| z32d_ut.ibs * IBIS 5.0 Model
| 16Gb DDR4 SDRAM - Die Revision "E"
| This Model is valid for Ultra-High Automotive Temperature Range -40C<=Tc<=125C
| Valid for DDR4-1600/1866/2133/2400/2666/2933/3200 operation
| Models *_3200 are applicable for speed grade 3200 Mbps (-062) and below
| Part Number   VDD/VDDQ   Architecture   Package
| MT40A4G4JE   1.2V/1.2V   4Gb   x  4   78-Ball FBGA
| MT40A2G8JE   1.2V/1.2V   2Gb   x  8   78-Ball FBGA
| MT40A1G16KH   1.2V/1.2V   1Gb   x 16   96-Ball FBGA
| MT40A4G4Z32D   1.2V/1.2V   4Gb   x 4   (Bare Die, x4)
| MT40A2G8Z32D   1.2V/1.2V   2Gb   x 8   (Bare Die, x8)
| MT40A1G16Z32D   1.2V/1.2V   1Gb   x 16   (Bare Die, x16)
[IBIS Ver]   5.0
[File Name]   z32d_ut.ibs
[Date]   5/19/2021
[File Rev]   2.4.2
[Source]   From silicon level SPICE model at Micron Technology, Inc.
   For support contact your local Micron FAE/Sales contacts
   (more information at https://www.micron.com/support/sales-network)
[Notes]   Revision History:
   Rev 2.4.2: 5/19/2021
   - Updated Part Numbers and Package Codes for Automotive parts
   Rev 2.4.1: 11/30/2020
   - Fixed submodels used for ODT models
   Rev 2.4: 11/16/2020
   - Simulated with new device models
   - Added Automotive and Industrial temperature ranges
   Rev 2.3: 9/11/2020
   - Updated c_comp with 8/19/2020 IOCAP measurements
   - Added x16 package model (9/2/2020 data)
   Rev 2.2: 8/4/2020
   - Updated c_comp with 6/25/2020 IOCAP measurements
   - Updated x4 and x8 package configuration based on 7/30/2020 data
   Rev 2.0: 8/27/2019
   - Matched IV curves with 8/22/2019 Z32D silicon measurements
   Rev 0.3: 8/9/2019
   - Component RLC data and Sparse Matrix Package Model updated with
   z32d specific data
   - Added x16 package model.
   Rev 0.2: 8/2/2019
   - Simulations ran with z32d SPF netlists.
   - C_comp values updated with 5/6/2019 z32d iocap data.
   - PU/PD trims similar with z22a trims.
   - Component RLC data and Sparse Matrix Package Model borrowed from z23c.
   - Will get z32d specific trims and package data in a couple of weeks.
   Rev 0.1: 5/17/2019
   - Initial pre-silicon model
   - All models were created from z32c SPF netlists.
   Notes:
   - The DQ_IN_ODT* models contain assumed input thresholds,
   the actual threshold values will depend on the VREFDQ
   level set by training
   - This IBIS file uses the Submodel keyword to model the
   DDR4 On-die Termination(ODT) characteristics.
   - The C_comp value in the DQ I/O model is set to match the
   input state of the DQ I/O as measured from the HSPICE model.
   The C_comp value decreases in the DQ/DQS Input ODT models.
   - L_pin values in the Pin sections are loop inductance and
   include the mutual inductance to appropriate POWER/GND
   return paths.  POWER/GND parasitics are modeled in the
   Package Models.
   - Typ and slow corner V-t curves in the following DQ* models
   are shifted relative to strong corner V-t curve
   to contain all 3 corners within appropriate V-t window
   Models   Typ   Slow   V-t duration
   DQ*_34_3200   -100ps   -240ps   440ps
   DQ*_40_3200   -100ps   -240ps   440ps
   DQ*_48_3200   -100ps   -240ps   440ps
   ALERT_3200   -40ps   -100ps   500ps
   - Due to the shift in typ and slow corner, the V-t curves
   may overlap each other. This does not effect the accuracy
   of the IBIS data.
   - The NF_INPUT Model is for Non-functioning INPUT pins in the
   x8 package
   - The NF_DQ Model is for Non-functioning DQ pins in the
   x4 package
   See Micron IBIS Model Quality Report and Quality Checklist
   for full IQ details
[Disclaimer]  This software code and all associated documentation, comments
   or other information (collectively "Software") is provided
   "AS IS" without warranty of any kind. MICRON TECHNOLOGY, INC.
   ("MTI") EXPRESSLY DISCLAIMS ALL WARRANTIES EXPRESS OR IMPLIED,
   INCLUDING BUT NOT LIMITED TO, NONINFRINGEMENT OF THIRD PARTY
   RIGHTS, AND ANY IMPLIED WARRANTIES OF MERCHANTABILITY OR
   FITNESS FOR ANY PARTICULAR PURPOSE. MTI DOES NOT WARRANT THAT
   THE SOFTWARE WILL MEET YOUR REQUIREMENTS, OR THAT THE
   OPERATION OF THE SOFTWARE WILL BE UNINTERRUPTED OR ERROR-FREE.
   FURTHERMORE, MTI DOES NOT MAKE ANY REPRESENTATIONS REGARDING
   THE USE OR THE RESULTS OF THE USE OF THE SOFTWARE IN TERMS OF
   ITS CORRECTNESS, ACCURACY, RELIABILITY, OR OTHERWISE. THE
   ENTIRE RISK ARISING OUT OF USE OR PERFORMANCE OF THE SOFTWARE
   REMAINS WITH YOU. IN NO EVENT SHALL MTI, ITS AFFILIATED
   COMPANIES OR THEIR SUPPLIERS BE LIABLE FOR ANY DIRECT,
   INDIRECT, CONSEQUENTIAL, INCIDENTAL, OR SPECIAL DAMAGES
   (INCLUDING, WITHOUT LIMITATION, DAMAGES FOR LOSS OF PROFITS,
   BUSINESS INTERRUPTION, OR LOSS OF INFORMATION) ARISING OUT OF
   YOUR USE OF OR INABILITY TO USE THE SOFTWARE, EVEN IF MTI HAS
   BEEN ADVISED OF THE POSSIBILITY OF SUCH DAMAGES. Because some
   jurisdictions prohibit the exclusion or limitation of
   liability for consequential or incidental damages, the above
   limitation may not apply to you.
[Copyright]   Copyright 2021 Micron Technology, Inc. All rights reserved.
| COMPONENT: MT40A4G4JE (78-Ball FBGA, x4)
[Component]   MT40A4G4JE
[Package Model] z32d_78ball_pkg
[Manufacturer]  Micron Technology,Inc.
[Package]
|   typ   min   max
R_pkg   0.456   0.390   0.524
L_pkg   1.988nH   1.619nH   2.308nH
C_pkg   0.525pF   0.416pF   0.832pF
[Pin]   signal_name   model_name   R_pin   L_pin   C_pin   | TD_pin(ps)   Z_pin
A1   VDD   POWER
A2   VSSQ   GND
A3   NF   NF_DQ   0.489   1.750nH   0.545pF   | 30.894   56.647
A7   NF   NF_DQ   0.511   1.874nH   0.589pF   | 33.231   56.384
A8   VSSQ   GND
A9   VSS   GND
B1   VPP   POWER
B2   VDDQ   POWER
B3   DQS_c   DQS   0.486   1.773nH   0.525pF   | 30.517   58.085
B7   DQ1   DQ   0.501   1.800nH   0.562pF   | 31.820   56.584
B8   VDDQ   POWER
B9   ZQ   NC
C1   VDDQ   POWER
C2   DQ0   DQ   0.474   1.679nH   0.533pF   | 29.920   56.108
C3   DQS_t   DQS   0.476   1.822nH   0.496pF   | 30.052   60.618
C7   VDD   POWER
C8   VSS   GND
C9   VDDQ   POWER
D1   VSS   GND
D2   NC   NC
D3   DQ2   DQ   0.472   1.854nH   0.500pF   | 30.432   60.921
D7   DQ3   DQ   0.507   1.896nH   0.570pF   | 32.871   57.672
D8   NC   NC
D9   VSS   GND
E1   VSSL   GND
E2   VDDQ   POWER
E3   NC   NC
E7   NC   NC
E8   VDDQ   POWER
E9   VSS   GND
F1   VDDL   POWER
F2   NC   NC
F3   ODT   INPUT   0.411   1.925nH   0.513pF   | 31.424   61.251
F7   CK_t   CLKIN   0.443   1.798nH   0.465pF   | 28.925   62.150
F8   CK_c   CLKIN   0.444   1.736nH   0.480pF   | 28.878   60.124
F9   VDD   POWER
G1   VSS   GND
G2   NC   NC
G3   CKE   INPUT   0.409   1.964nH   0.404pF   | 28.176   69.706
G7   CS_n   INPUT   0.431   1.908nH   0.432pF   | 28.718   66.430
G8   NC   NC
G9   TEN   INPUT   0.383   1.791nH   0.817pF   | 38.251   46.825
H1   VDD   POWER
H2   WE_n_A14   INPUT   0.418   2.109nH   0.449pF   | 30.769   68.534
H3   ACT_n   INPUT   0.417   1.961nH   0.401pF   | 28.060   69.898
H7   CAS_n_A15   INPUT   0.424   2.012nH   0.494pF   | 31.537   63.804
H8   RAS_n_A16   INPUT   0.454   2.168nH   0.498pF   | 32.847   66.005
H9   VSS   GND
J1   VREFCA   POWER
J2   BG0   INPUT   0.413   2.000nH   0.463pF   | 30.442   65.692
J3   A10   INPUT   0.419   1.998nH   0.414pF   | 28.764   69.471
J7   A12_BC_n   INPUT   0.445   2.033nH   0.493pF   | 31.668   64.200
J8   BG1   INPUT   0.416   2.015nH   0.444pF   | 29.919   67.359
J9   VDD   POWER
K1   VSS   GND
K2   BA0   INPUT   0.411   1.987nH   0.489pF   | 31.161   63.771
K3   A4   INPUT   0.439   2.097nH   0.466pF   | 31.268   67.077
K7   A3   INPUT   0.464   2.043nH   0.494pF   | 31.777   64.281
K8   BA1   INPUT   0.447   1.943nH   0.510pF   | 31.478   61.723
K9   VSS   GND
L1   RESET_n   INPUT   0.362   1.895nH   0.778pF   | 38.392   49.358
L2   A6   INPUT   0.451   2.165nH   0.503pF   | 33.004   65.598
L3   A0   INPUT   0.424   2.147nH   0.458pF   | 31.371   68.448
L7   A1   INPUT   0.468   2.166nH   0.437pF   | 30.762   70.406
L8   A5   INPUT   0.474   2.194nH   0.528pF   | 34.017   64.487
L9   ALERT_n   ALERT   0.367   1.782nH   0.744pF   | 36.422   48.927
M1   VDD   POWER
M2   A8   INPUT   0.409   2.072nH   0.479pF   | 31.515   65.733
M3   A2   INPUT   0.427   2.141nH   0.444pF   | 30.824   69.466
M7   A9   INPUT   0.470   2.288nH   0.481pF   | 33.168   68.967
M8   A7   INPUT   0.447   2.196nH   0.519pF   | 33.774   65.017
M9   VPP   POWER
N1   VSS   GND
N2   A11   INPUT   0.441   2.192nH   0.480pF   | 32.443   67.581
N3   PARITY   INPUT   0.378   1.641nH   0.470pF   | 27.766   59.114
N7   A17   INPUT   0.407   1.906nH   0.476pF   | 30.114   63.296
N8   A13   INPUT   0.469   2.299nH   0.563pF   | 35.991   63.889
N9   VDD   POWER
|***********************PIN MAPPING*****************************************
[Pin Mapping]   pulldown_ref   pullup_ref   gnd_clamp_ref   power_clamp_ref ext_ref
A1   NC   VDD
A2   VSS   NC
A3   NC   NC   VSS   VDDQ
A7   NC   NC   VSS   VDDQ
A8   VSS   NC
A9   VSS   NC
B1   NC   VPP
B2   NC   VDDQ
B3   VSS   VDDQ   VSS   VDDQ
B7   VSS   VDDQ   VSS   VDDQ
B8   NC   VDDQ
B9   NC   NC
C1   NC   VDDQ
C2   VSS   VDDQ   VSS   VDDQ
C3   VSS   VDDQ   VSS   VDDQ
C7   NC   VDD
C8   VSS   NC
C9   NC   VDDQ
D1   VSS   NC
D2   NC   NC
D3   VSS   VDDQ   VSS   VDDQ
D7   VSS   VDDQ   VSS   VDDQ
D8   NC   NC
D9   VSS   NC
E1   VSSL   NC
E2   NC   VDDQ
E3   NC   NC
E7   NC   NC
E8   NC   VDDQ
E9   VSS   NC
F1   NC   VDDL
F2   NC   NC
F3   NC   NC   VSS   VDD
F7   NC   NC   VSS   VDD
F8   NC   NC   VSS   VDD
F9   NC   VDD
G1   VSS   NC
G2   NC   NC
G3   NC   NC   VSS   VDD
G7   NC   NC   VSS   VDD
G8   NC   NC
G9   NC   NC   VSS   VDD
H1   NC   VDD
H2   NC   NC   VSS   VDD
H3   NC   NC   VSS   VDD
H7   NC   NC   VSS   VDD
H8   NC   NC   VSS   VDD
H9   VSS   NC
J1   NC   VREFCA
J2   NC   NC   VSS   VDD
J3   NC   NC   VSS   VDD
J7   NC   NC   VSS   VDD
J8   NC   NC   VSS   VDD
J9   NC   VDD
K1   VSS   NC
K2   NC   NC   VSS   VDD
K3   NC   NC   VSS   VDD
K7   NC   NC   VSS   VDD
K8   NC   NC   VSS   VDD
K9   VSS   NC
L1   NC   NC   VSS   VDD
L2   NC   NC   VSS   VDD
L3   NC   NC   VSS   VDD
L7   NC   NC   VSS   VDD
L8   NC   NC   VSS   VDD
L9   VSS   VDDQ   VSS   VDDQ
M1   NC   VDD
M2   NC   NC   VSS   VDD
M3   NC   NC   VSS   VDD
M7   NC   NC   VSS   VDD
M8   NC   NC   VSS   VDD
M9   NC   VPP
N1   VSS   NC
N2   NC   NC   VSS   VDD
N3   NC   NC   VSS   VDD
N7   NC   NC   VSS   VDD
N8   NC   NC   VSS   VDD
N9   NC   VDD
|**********************DIFF PIN*********************************************
[Diff_pin]   inv_pin   vdiff   tdelay_typ   tdelay_min   tdelay_max
   C3   B3   0.000V   0ns   NA   NA
   F7   F8   0.250V   0ns   NA   NA
| COMPONENT: MT40A2G8JE (78-Ball FBGA, x8)
[Component]   MT40A2G8JE
[Package Model] z32d_78ball_pkg
[Manufacturer]  Micron Technology,Inc.
[Package]
|   typ   min   max
R_pkg   0.460   0.390   0.530
L_pkg   1.971nH   1.619nH   2.308nH
C_pkg   0.530pF   0.416pF   0.832pF
[Pin]   signal_name   model_name   R_pin   L_pin   C_pin   | TD_pin(ps)   Z_pin
A1   VDD   POWER
A2   VSSQ   GND
A3   TDQS_c   TDQS   0.489   1.750nH   0.545pF   | 30.894   56.647
A7   DM_n_DBI_n_TDQS_t DM_DBI_TDQS   0.511   1.874nH   0.589pF   | 33.231   56.384
A8   VSSQ   GND
A9   VSS   GND
B1   VPP   POWER
B2   VDDQ   POWER
B3   DQS_c   DQS   0.486   1.773nH   0.525pF   | 30.517   58.085
B7   DQ1   DQ   0.501   1.800nH   0.562pF   | 31.820   56.584
B8   VDDQ   POWER
B9   ZQ   NC
C1   VDDQ   POWER
C2   DQ0   DQ   0.474   1.679nH   0.533pF   | 29.920   56.108
C3   DQS_t   DQS   0.476   1.822nH   0.496pF   | 30.052   60.618
C7   VDD   POWER
C8   VSS   GND
C9   VDDQ   POWER
D1   VSS   GND
D2   DQ4   DQ   0.474   1.688nH   0.550pF   | 30.479   55.389
D3   DQ2   DQ   0.472   1.854nH   0.500pF   | 30.432   60.921
D7   DQ3   DQ   0.507   1.896nH   0.570pF   | 32.871   57.672
D8   DQ5   DQ   0.506   1.785nH   0.563pF   | 31.711   56.288
D9   VSS   GND
E1   VSSL   GND
E2   VDDQ   POWER
E3   DQ6   DQ   0.457   1.712nH   0.527pF   | 30.045   56.978
E7   DQ7   DQ   0.514   1.980nH   0.591pF   | 34.226   57.866
E8   VDDQ   POWER
E9   VSS   GND
F1   VDDL   POWER
F2   NC   NC
F3   ODT   INPUT   0.411   1.925nH   0.513pF   | 31.424   61.251
F7   CK_t   CLKIN   0.443   1.798nH   0.465pF   | 28.925   62.150
F8   CK_c   CLKIN   0.444   1.736nH   0.480pF   | 28.878   60.124
F9   VDD   POWER
G1   VSS   GND
G2   NC   NC
G3   CKE   INPUT   0.409   1.964nH   0.404pF   | 28.176   69.706
G7   CS_n   INPUT   0.431   1.908nH   0.432pF   | 28.718   66.430
G8   NC   NC
G9   TEN   INPUT   0.383   1.791nH   0.817pF   | 38.251   46.825
H1   VDD   POWER
H2   WE_n_A14   INPUT   0.418   2.109nH   0.449pF   | 30.769   68.534
H3   ACT_n   INPUT   0.417   1.961nH   0.401pF   | 28.060   69.898
H7   CAS_n_A15   INPUT   0.424   2.012nH   0.494pF   | 31.537   63.804
H8   RAS_n_A16   INPUT   0.454   2.168nH   0.498pF   | 32.847   66.005
H9   VSS   GND
J1   VREFCA   POWER
J2   BG0   INPUT   0.413   2.000nH   0.463pF   | 30.442   65.692
J3   A10   INPUT   0.419   1.998nH   0.414pF   | 28.764   69.471
J7   A12_BC_n   INPUT   0.445   2.033nH   0.493pF   | 31.668   64.200
J8   BG1   INPUT   0.416   2.015nH   0.444pF   | 29.919   67.359
J9   VDD   POWER
K1   VSS   GND
K2   BA0   INPUT   0.411   1.987nH   0.489pF   | 31.161   63.771
K3   A4   INPUT   0.439   2.097nH   0.466pF   | 31.268   67.077
K7   A3   INPUT   0.464   2.043nH   0.494pF   | 31.777   64.281
K8   BA1   INPUT   0.447   1.943nH   0.510pF   | 31.478   61.723
K9   VSS   GND
L1   RESET_n   INPUT   0.362   1.895nH   0.778pF   | 38.392   49.358
L2   A6   INPUT   0.451   2.165nH   0.503pF   | 33.004   65.598
L3   A0   INPUT   0.424   2.147nH   0.458pF   | 31.371   68.448
L7   A1   INPUT   0.468   2.166nH   0.437pF   | 30.762   70.406
L8   A5   INPUT   0.474   2.194nH   0.528pF   | 34.017   64.487
L9   ALERT_n   ALERT   0.367   1.782nH   0.744pF   | 36.422   48.927
M1   VDD   POWER
M2   A8   INPUT   0.409   2.072nH   0.479pF   | 31.515   65.733
M3   A2   INPUT   0.427   2.141nH   0.444pF   | 30.824   69.466
M7   A9   INPUT   0.470   2.288nH   0.481pF   | 33.168   68.967
M8   A7   INPUT   0.447   2.196nH   0.519pF   | 33.774   65.017
M9   VPP   POWER
N1   VSS   GND
N2   A11   INPUT   0.441   2.192nH   0.480pF   | 32.443   67.581
N3   PARITY   INPUT   0.378   1.641nH   0.470pF   | 27.766   59.114
N7   A17   NF_INPUT   0.407   1.906nH   0.476pF   | 30.114   63.296
N8   A13   INPUT   0.469   2.299nH   0.563pF   | 35.991   63.889
N9   VDD   POWER
|***********************PIN MAPPING*****************************************
[Pin Mapping]   pulldown_ref   pullup_ref   gnd_clamp_ref   power_clamp_ref ext_ref
A1   NC   VDD
A2   VSS   NC
A3   VSS   VDDQ   VSS   VDDQ
A7   VSS   VDDQ   VSS   VDDQ
A8   VSS   NC
A9   VSS   NC
B1   NC   VPP
B2   NC   VDDQ
B3   VSS   VDDQ   VSS   VDDQ
B7   VSS   VDDQ   VSS   VDDQ
B8   NC   VDDQ
B9   NC   NC
C1   NC   VDDQ
C2   VSS   VDDQ   VSS   VDDQ
C3   VSS   VDDQ   VSS   VDDQ
C7   NC   VDD
C8   VSS   NC
C9   NC   VDDQ
D1   VSS   NC
D2   VSS   VDDQ   VSS   VDDQ
D3   VSS   VDDQ   VSS   VDDQ
D7   VSS   VDDQ   VSS   VDDQ
D8   VSS   VDDQ   VSS   VDDQ
D9   VSS   NC
E1   VSSL   NC
E2   NC   VDDQ
E3   VSS   VDDQ   VSS   VDDQ
E7   VSS   VDDQ   VSS   VDDQ
E8   NC   VDDQ
E9   VSS   NC
F1   NC   VDDL
F2   NC   NC
F3   NC   NC   VSS   VDD
F7   NC   NC   VSS   VDD
F8   NC   NC   VSS   VDD
F9   NC   VDD
G1   VSS   NC
G2   NC   NC
G3   NC   NC   VSS   VDD
G7   NC   NC   VSS   VDD
G8   NC   NC
G9   NC   NC   VSS   VDD
H1   NC   VDD
H2   NC   NC   VSS   VDD
H3   NC   NC   VSS   VDD
H7   NC   NC   VSS   VDD
H8   NC   NC   VSS   VDD
H9   VSS   NC
J1   NC   VREFCA
J2   NC   NC   VSS   VDD
J3   NC   NC   VSS   VDD
J7   NC   NC   VSS   VDD
J8   NC   NC   VSS   VDD
J9   NC   VDD
K1   VSS   NC
K2   NC   NC   VSS   VDD
K3   NC   NC   VSS   VDD
K7   NC   NC   VSS   VDD
K8   NC   NC   VSS   VDD
K9   VSS   NC
L1   NC   NC   VSS   VDD
L2   NC   NC   VSS   VDD
L3   NC   NC   VSS   VDD
L7   NC   NC   VSS   VDD
L8   NC   NC   VSS   VDD
L9   VSS   VDDQ   VSS   VDDQ
M1   NC   VDD
M2   NC   NC   VSS   VDD
M3   NC   NC   VSS   VDD
M7   NC   NC   VSS   VDD
M8   NC   NC   VSS   VDD
M9   NC   VPP
N1   VSS   NC
N2   NC   NC   VSS   VDD
N3   NC   NC   VSS   VDD
N7   NC   NC   VSS   VDD
N8   NC   NC   VSS   VDD
N9   NC   VDD
|**********************DIFF PIN*********************************************
[Diff_pin]   inv_pin   vdiff   tdelay_typ   tdelay_min   tdelay_max
   C3   B3   0.000V   0ns   NA   NA
   F7   F8   0.250V   0ns   NA   NA
| COMPONENT: MT40A1G16KH (96-Ball FBGA, x16)
[Component]   MT40A1G16KH
[Package Model] z32d_96ball_pkg
[Manufacturer]  Micron Technology,Inc.
[Package]
|   typ   min   max
R_pkg   0.493   0.376   0.603
L_pkg   2.127nH   1.296nH   3.043nH
C_pkg   0.508pF   0.353pF   0.791pF
[Pin]   signal_name   model_name   R_pin   L_pin   C_pin   | TD_pin(ps)   Z_pin
A1   VDDQ   POWER
A2   VSSQ   GND
A3   DQ8   DQ   0.485   1.863nH   0.572pF   | 32.649   57.054
A7   UDQS_c   DQS   0.515   1.883nH   0.607pF   | 33.816   55.671
A8   VSSQ   GND
A9   VDDQ   POWER
B1   VPP   POWER
B2   VSS   GND
B3   VDD   POWER
B7   UDQS_t   DQS   0.516   1.973nH   0.597pF   | 34.324   57.471
B8   DQ9   DQ   0.514   1.965nH   0.559pF   | 33.151   59.270
B9   VDD   POWER
C1   VDDQ   POWER
C2   DQ12   DQ   0.488   1.847nH   0.515pF   | 30.844   59.889
C3   DQ10   DQ   0.482   1.869nH   0.566pF   | 32.513   57.487
C7   DQ11   DQ   0.513   1.889nH   0.545pF   | 32.101   58.855
C8   DQ13   DQ   0.522   1.989nH   0.555pF   | 33.225   59.871
C9   VSSQ   GND
D1   VDD   POWER
D2   VSSQ   GND
D3   DQ14   DQ   0.477   1.899nH   0.554pF   | 32.437   58.550
D7   DQ15   DQ   0.520   1.859nH   0.597pF   | 33.298   55.815
D8   VSSQ   GND
D9   VDDQ   POWER
E1   VSS   GND
E2   UDM_n_UDBI_n   DM_DBI   0.487   1.699nH   0.581pF   | 31.427   54.054
E3   VSSQ   GND
E7   LDM_n_LDBI_n   DM_DBI   0.406   1.463nH   0.466pF   | 26.106   56.056
E8   VSSQ   GND
E9   VSS   GND
F1   VSSQ   GND
F2   VDDQ   POWER
F3   LDQS_c   DQS   0.376   1.314nH   0.441pF   | 24.072   54.582
F7   DQ1   DQ   0.404   1.440nH   0.445pF   | 25.315   56.886
F8   VDDQ   POWER
F9   ZQ   NC
G1   VDDQ   POWER
G2   DQ0   DQ   0.374   1.462nH   0.410pF   | 24.490   59.711
G3   LDQS_t   DQS   0.384   1.347nH   0.420pF   | 23.781   56.647
G7   VDD   POWER
G8   VSS   GND
G9   VDDQ   POWER
H1   VSSQ   GND
H2   DQ4   DQ   0.376   1.434nH   0.432pF   | 24.905   57.594
H3   DQ2   DQ   0.380   1.349nH   0.413pF   | 23.618   57.141
H7   DQ3   DQ   0.405   1.482nH   0.460pF   | 26.107   56.750
H8   DQ5   DQ   0.404   1.507nH   0.422pF   | 25.207   59.793
H9   VSSQ   GND
J1   VDDL   POWER
J2   VDDQ   POWER
J3   DQ6   DQ   0.381   1.338nH   0.426pF   | 23.880   56.023
J7   DQ7   DQ   0.407   1.439nH   0.455pF   | 25.582   56.260
J8   VDDQ   POWER
J9   VDD   POWER
K1   VSSL   GND
K2   CKE   INPUT   0.382   1.804nH   0.414pF   | 27.332   65.986
K3   ODT   INPUT   0.378   1.618nH   0.365pF   | 24.289   66.601
K7   CK_t   CLKIN   0.433   1.750nH   0.426pF   | 27.313   64.067
K8   CK_c   CLKIN   0.439   1.738nH   0.484pF   | 28.992   59.948
K9   VSS   GND
L1   VDD   POWER
L2   WE_n_A14   INPUT   0.529   2.529nH   0.546pF   | 37.143   68.080
L3   ACT_n   INPUT   0.505   2.402nH   0.530pF   | 35.678   67.312
L7   CS_n   INPUT   0.421   1.808nH   0.417pF   | 27.443   65.875
L8   RAS_n   INPUT   0.572   2.697nH   0.621pF   | 40.942   65.885
L9   VDD   POWER
M1   VREFCA   POWER
M2   BG0   INPUT   0.522   2.644nH   0.543pF   | 37.876   69.816
M3   A10   INPUT   0.519   2.313nH   0.496pF   | 33.857   68.326
M7   A12_BC_n   INPUT   0.539   2.480nH   0.453pF   | 33.501   74.022
M8   CAS_n_A15   INPUT   0.559   2.644nH   0.526pF   | 37.298   70.901
M9   VSS   GND
N1   VSS   GND
N2   BA0   INPUT   0.522   2.594nH   0.540pF   | 37.444   69.282
N3   A4   INPUT   0.531   2.537nH   0.487pF   | 35.143   72.181
N7   A3   INPUT   0.543   2.444nH   0.502pF   | 35.013   69.814
N8   BA1   INPUT   0.546   2.611nH   0.546pF   | 37.766   69.125
N9   TEN   INPUT   0.567   2.612nH   0.631pF   | 40.595   64.341
P1   RESET_n   INPUT   0.454   2.115nH   0.829pF   | 41.867   50.528
P2   A6   INPUT   0.531   2.622nH   0.530pF   | 37.272   70.340
P3   A0   INPUT   0.523   2.599nH   0.517pF   | 36.644   70.932
P7   A1   INPUT   0.543   2.675nH   0.533pF   | 37.751   70.847
P8   A5   INPUT   0.573   2.741nH   0.573pF   | 39.614   69.193
P9   ALERT_n   ALERT   0.599   3.051nH   0.692pF   | 45.952   66.397
R1   VDD   POWER
R2   A8   INPUT   0.546   2.743nH   0.576pF   | 39.737   69.023
R3   A2   INPUT   0.528   2.627nH   0.560pF   | 38.368   68.463
R7   A9   INPUT   0.557   2.804nH   0.559pF   | 39.575   70.850
R8   A7   INPUT   0.579   2.925nH   0.603pF   | 41.984   69.669
R9   VPP   POWER
T1   VSS   GND
T2   A11   INPUT   0.549   2.659nH   0.625pF   | 40.777   65.214
T3   PARITY   INPUT   0.548   2.315nH   0.632pF   | 38.265   60.507
T7   A17   INPUT   0.571   2.752nH   0.596pF   | 40.507   67.946
T8   A13   INPUT   0.570   2.905nH   0.607pF   | 41.999   69.167
T9   VDD   POWER
|***********************PIN MAPPING*****************************************
[Pin Mapping]   pulldown_ref   pullup_ref   gnd_clamp_ref   power_clamp_ref ext_ref
A1   NC   VDDQ
A2   VSS   NC
A3   VSS   VDDQ   VSS   VDDQ
A7   VSS   VDDQ   VSS   VDDQ
A8   VSS   NC
A9   NC   VDDQ
B1   NC   VPP
B2   VSS   NC
B3   NC   VDD
B7   VSS   VDDQ   VSS   VDDQ
B8   VSS   VDDQ   VSS   VDDQ
B9   NC   VDD
C1   NC   VDDQ
C2   VSS   VDDQ   VSS   VDDQ
C3   VSS   VDDQ   VSS   VDDQ
C7   VSS   VDDQ   VSS   VDDQ
C8   VSS   VDDQ   VSS   VDDQ
C9   VSS   NC
D1   NC   VDD
D2   VSS   NC
D3   VSS   VDDQ   VSS   VDDQ
D7   VSS   VDDQ   VSS   VDDQ
D8   VSS   NC
D9   NC   VDDQ
E1   VSS   NC
E2   VSS   VDDQ   VSS   VDDQ
E3   VSS   NC
E7   VSS   VDDQ   VSS   VDDQ
E8   VSS   NC
E9   VSS   NC
F1   VSS   NC
F2   NC   VDDQ
F3   VSS   VDDQ   VSS   VDDQ
F7   VSS   VDDQ   VSS   VDDQ
F8   NC   VDDQ
F9   NC   NC
G1   NC   VDDQ
G2   VSS   VDDQ   VSS   VDDQ
G3   VSS   VDDQ   VSS   VDDQ
G7   NC   VDD
G8   VSS   NC
G9   NC   VDDQ
H1   VSS   NC
H2   VSS   VDDQ   VSS   VDDQ
H3   VSS   VDDQ   VSS   VDDQ
H7   VSS   VDDQ   VSS   VDDQ
H8   VSS   VDDQ   VSS   VDDQ
H9   VSS   NC
J1   NC   VDDL
J2   NC   VDDQ
J3   VSS   VDDQ   VSS   VDDQ
J7   VSS   VDDQ   VSS   VDDQ
J8   NC   VDDQ
J9   NC   VDD
K1   VSSL   NC
K2   NC   NC   VSS   VDD
K3   NC   NC   VSS   VDD
K7   NC   NC   VSS   VDD
K8   NC   NC   VSS   VDD
K9   VSS   NC
L1   NC   VDD
L2   NC   NC   VSS   VDD
L3   NC   NC   VSS   VDD
L7   NC   NC   VSS   VDD
L8   NC   NC   VSS   VDD
L9   NC   VDD
M1   NC   VREFCA
M2   NC   NC   VSS   VDD
M3   NC   NC   VSS   VDD
M7   NC   NC   VSS   VDD
M8   NC   NC   VSS   VDD
M9   VSS   NC
N1   VSS   NC
N2   NC   NC   VSS   VDD
N3   NC   NC   VSS   VDD
N7   NC   NC   VSS   VDD
N8   NC   NC   VSS   VDD
N9   NC   NC   VSS   VDD
P1   NC   NC   VSS   VDD
P2   NC   NC   VSS   VDD
P3   NC   NC   VSS   VDD
P7   NC   NC   VSS   VDD
P8   NC   NC   VSS   VDD
P9   VSS   VDDQ   VSS   VDDQ
R1   NC   VDD
R2   NC   NC   VSS   VDD
R3   NC   NC   VSS   VDD
R7   NC   NC   VSS   VDD
R8   NC   NC   VSS   VDD
R9   NC   VPP
T1   VSS   NC
T2   NC   NC   VSS   VDD
T3   NC   NC   VSS   VDD
T7   NC   NC   VSS   VDD
T8   NC   NC   VSS   VDD
T9   NC   VDD
|**********************DIFF PIN*********************************************
[Diff_pin]   inv_pin   vdiff   tdelay_typ   tdelay_min   tdelay_max
   B7   A7   0.000V   0ns   NA   NA
   G3   F3   0.000V   0ns   NA   NA
   K7   K8   0.250V   0ns   NA   NA
| COMPONENT: MT40A4G4Z32D (Bare Die, x4)
[Component]   MT40A4G4Z32D
[Manufacturer]  Micron Technology,Inc.
[Package]
|   typ   min   max
R_pkg   0.001   0.001   0.001
L_pkg   0.001nH   0.001nH   0.001nH
C_pkg   0.001pF   0.001pF   0.001pF
[Pin]   signal_name   model_name   R_pin   L_pin   C_pin
1   VSS   GND
2   VDD   POWER
3   VPP   POWER
4   NC   NC
5   VDDQ   POWER
6   NC   NC
7   VSS   GND
8   NC   NC
9   VDDQ   POWER
10   NC   NC
11   VSS   GND
12   NC   NC
13   VDDQ   POWER
14   NC   NC
15   VSS   GND
16   VDDQ   POWER
17   VDD   POWER
18   VSS   GND
19   NC   NC
20   VDDQ   POWER
21   NC   NC
22   VSS   GND
23   NC   NC
24   VDDQ   POWER
25   NF   NF_DQ
26   VSS   GND
27   NC   NC
28   VDDQ   POWER
29   NC   NC
30   VSS   GND
31   VDD   POWER
32   VSS   GND
33   ZQ   NC
34   VDDQ   POWER
35   DQS_c   DQS
36   VSS   GND
37   DQS_t   DQS
38   VDDQ   POWER
39   NF   NF_DQ
40   VSS   GND
41   DQ1   DQ
42   VDDQ   POWER
43   DQ3   DQ
44   VSS   GND
45   DQ0   DQ
46   VDDQ   POWER
47   DQ2   DQ
48   VSS   GND
49   VDDQ   POWER
50   VDD   POWER
51   VSS   GND
52   DQ5   NC
53   VDDQ   POWER
54   DQ7   NC
55   VSS   GND
56   DQ4   NC
57   VDDQ   POWER
58   DQ6   NC
59   VSS   GND
60   VDD   POWER
61   VSS   GND
62   VDD   POWER
63   VDDL   POWER
64   VSS   GND
65   CK_t   CLKIN
66   CK_c   CLKIN
67   VSS   GND
68   VDD   POWER
69   ODT   INPUT
70   CS_n   INPUT
71   NC   NC
72   CKE   INPUT
73   NC   NC
74   RAS_n_A16   INPUT
75   WE_n_A14   INPUT
76   CAS_n_A15   INPUT
77   ACT_n   INPUT
78   BG1   INPUT
79   A10   INPUT
80   A12_BC_n   INPUT
81   BG0   INPUT
82   BA1   INPUT
83   BA0   INPUT
84   VSS   GND
85   VREFCA   POWER
86   VDD   POWER
87   A3   INPUT
88   A4   INPUT
89   A5   INPUT
90   A0   INPUT
91   A1   INPUT
92   A6   INPUT
93   A7   INPUT
94   A8   INPUT
95   A9   INPUT
96   A2   INPUT
97   A13   INPUT
98   A11   INPUT
99   A17   INPUT
100   PARITY   INPUT
101   VSS   GND
102   VDD   POWER
103   TEN   INPUT
104   RESET_n   INPUT
105   ALERT_n   ALERT
106   NC   NC
107   NC   NC
108   NC   NC
109   VPP   POWER
110   VDD   POWER
111   VSS   GND
112   NC   NC
|**********************DIFF PIN*********************************************
[Diff_pin]   inv_pin   vdiff   tdelay_typ   tdelay_min   tdelay_max
   37   35   0.000V   0ns   NA   NA
   65   66   0.250V   0ns   NA   NA
| COMPONENT: MT40A2G8Z32D (Bare Die, x8)
[Component]   MT40A2G8Z32D
[Manufacturer]  Micron Technology,Inc.
[Package]
|   typ   min   max
R_pkg   0.001   0.001   0.001
L_pkg   0.001nH   0.001nH   0.001nH
C_pkg   0.001pF   0.001pF   0.001pF
[Pin]   signal_name   model_name   R_pin   L_pin   C_pin
1   VSS   GND
2   VDD   POWER
3   VPP   POWER
4   NC   NC
5   VDDQ   POWER
6   NC   NC
7   VSS   GND
8   NC   NC
9   VDDQ   POWER
10   NC   NC
11   VSS   GND
12   NC   NC
13   VDDQ   POWER
14   NC   NC
15   VSS   GND
16   VDDQ   POWER
17   VDD   POWER
18   VSS   GND
19   NC   NC
20   VDDQ   POWER
21   NC   NC
22   VSS   GND
23   NC   NC
24   VDDQ   POWER
25   TDQS_c   TDQS
26   VSS   GND
27   NC   NC
28   VDDQ   POWER
29   NC   NC
30   VSS   GND
31   VDD   POWER
32   VSS   GND
33   ZQ   NC
34   VDDQ   POWER
35   DQS_c   DQS
36   VSS   GND
37   DQS_t   DQS
38   VDDQ   POWER
39   DM_n_DBI_n_TDQS_t   DM_DBI_TDQS
40   VSS   GND
41   DQ1   DQ
42   VDDQ   POWER
43   DQ3   DQ
44   VSS   GND
45   DQ0   DQ
46   VDDQ   POWER
47   DQ2   DQ
48   VSS   GND
49   VDDQ   POWER
50   VDD   POWER
51   VSS   GND
52   DQ5   DQ
53   VDDQ   POWER
54   DQ7   DQ
55   VSS   GND
56   DQ4   DQ
57   VDDQ   POWER
58   DQ6   DQ
59   VSS   GND
60   VDD   POWER
61   VSS   GND
62   VDD   POWER
63   VDDL   POWER
64   VSS   GND
65   CK_t   CLKIN
66   CK_c   CLKIN
67   VSS   GND
68   VDD   POWER
69   ODT   INPUT
70   CS_n   INPUT
71   NC   NC
72   CKE   INPUT
73   NC   NC
74   RAS_n_A16   INPUT
75   WE_n_A14   INPUT
76   CAS_n_A15   INPUT
77   ACT_n   INPUT
78   BG1   INPUT
79   A10   INPUT
80   A12_BC_n   INPUT
81   BG0   INPUT
82   BA1   INPUT
83   BA0   INPUT
84   VSS   GND
85   VREFCA   POWER
86   VDD   POWER
87   A3   INPUT
88   A4   INPUT
89   A5   INPUT
90   A0   INPUT
91   A1   INPUT
92   A6   INPUT
93   A7   INPUT
94   A8   INPUT
95   A9   INPUT
96   A2   INPUT
97   A13   INPUT
98   A11   INPUT
99   A17   NF_INPUT
100   PARITY   INPUT
101   VSS   GND
102   VDD   POWER
103   TEN   INPUT
104   RESET_n   INPUT
105   ALERT_n   ALERT
106   NC   NC
107   NC   NC
108   NC   NC
109   VPP   POWER
110   VDD   POWER
111   VSS   GND
112   NC   NC
|**********************DIFF PIN*********************************************
[Diff_pin]   inv_pin   vdiff   tdelay_typ   tdelay_min   tdelay_max
   37   35   0.000V   0ns   NA   NA
   65   66   0.250V   0ns   NA   NA
| COMPONENT: MT40A1G16Z32D (Bare Die, x16)
[Component]   MT40A1G16Z32D
[Manufacturer]  Micron Technology,Inc.
[Package]
|   typ   min   max
R_pkg   0.001   0.001   0.001
L_pkg   0.001nH   0.001nH   0.001nH
C_pkg   0.001pF   0.001pF   0.001pF
[Pin]   signal_name   model_name   R_pin   L_pin   C_pin
1   VSS   GND
2   VDD   POWER
3   VPP   POWER
4   NC   NC
5   VDDQ   POWER
6   UDQS_c   DQS
7   VSS   GND
8   UDQS_t   DQS
9   VDDQ   POWER
10   DQ8   DQ
11   VSS   GND
12   DQ10   DQ
13   VDDQ   POWER
14   DQ12   DQ
15   VSS   GND
16   VDDQ   POWER
17   VDD   POWER
18   VSS   GND
19   DQ9   DQ
20   VDDQ   POWER
21   DQ11   DQ
22   VSS   GND
23   DQ14   DQ
24   VDDQ   POWER
25   UDM_n_UDBI_n   DM_DBI
26   VSS   GND
27   DQ13   DQ
28   VDDQ   POWER
29   DQ15   DQ
30   VSS   GND
31   VDD   POWER
32   VSS   GND
33   ZQ   NC
34   VDDQ   POWER
35   LDQS_c   DQS
36   VSS   GND
37   LDQS_t   DQS
38   VDDQ   POWER
39   LDM_n_LDBI_n   DM_DBI
40   VSS   GND
41   DQ1   DQ
42   VDDQ   POWER
43   DQ3   DQ
44   VSS   GND
45   DQ0   DQ
46   VDDQ   POWER
47   DQ2   DQ
48   VSS   GND
49   VDDQ   POWER
50   VDD   POWER
51   VSS   GND
52   DQ5   DQ
53   VDDQ   POWER
54   DQ7   DQ
55   VSS   GND
56   DQ4   DQ
57   VDDQ   POWER
58   DQ6   DQ
59   VSS   GND
60   VDD   POWER
61   VSS   GND
62   VDD   POWER
63   VDDL   POWER
64   VSS   GND
65   CK_t   CLKIN
66   CK_c   CLKIN
67   VSS   GND
68   VDD   POWER
69   ODT   INPUT
70   CS_n   INPUT
71   NC   NC
72   CKE   INPUT
73   NC   NC
74   RAS_n_A16   INPUT
75   WE_n_A14   INPUT
76   CAS_n_A15   INPUT
77   ACT_n   INPUT
78   BG1   INPUT
79   A10   INPUT
80   A12_BC_n   INPUT
81   BG0   INPUT
82   BA1   INPUT
83   BA0   INPUT
84   VSS   GND
85   VREFCA   POWER
86   VDD   POWER
87   A3   INPUT
88   A4   INPUT
89   A5   INPUT
90   A0   INPUT
91   A1   INPUT
92   A6   INPUT
93   A7   INPUT
94   A8   INPUT
95   A9   INPUT
96   A2   INPUT
97   A13   INPUT
98   A11   INPUT
99   A17   NF_INPUT
100   PARITY   INPUT
101   VSS   GND
102   VDD   POWER
103   TEN   INPUT
104   RESET_n   INPUT
105   ALERT_n   ALERT
106   NC   NC
107   NC   NC
108   NC   NC
109   VPP   POWER
110   VDD   POWER
111   VSS   GND
112   NC   NC
|**********************DIFF PIN*********************************************
[Diff_pin]   inv_pin   vdiff   tdelay_typ   tdelay_min   tdelay_max
   8   6   0.000V   0ns   NA   NA
   37   35   0.000V   0ns   NA   NA
   65   66   0.250V   0ns   NA   NA
|   Model Selector
[Model Selector] DQ
DQ_34_3200   34 Ohm Data I/O with no ODT, 1600-3200Mbps
DQ_40_3200   40 Ohm Data I/O with no ODT, 1600-3200Mbps
DQ_48_3200   48 Ohm Data I/O with no ODT, 1600-3200Mbps
DQ_IN_ODTOFF_3200  Data Input with no ODT, 1600-3200Mbps
DQ_IN_ODT34_3200   Data Input with 34ohm ODT, 1600-3200Mbps
DQ_IN_ODT40_3200   Data Input with 40ohm ODT, 1600-3200Mbps
DQ_IN_ODT48_3200   Data Input with 48ohm ODT, 1600-3200Mbps
DQ_IN_ODT60_3200   Data Input with 60ohm ODT, 1600-3200Mbps
DQ_IN_ODT80_3200   Data Input with 80ohm ODT, 1600-3200Mbps
DQ_IN_ODT120_3200  Data Input with 120ohm ODT, 1600-3200Mbps
DQ_IN_ODT240_3200  Data Input with 240ohm ODT, 1600-3200Mbps
[Model Selector] DQS
DQS_34_3200   34 Ohm Data Strobe I/O with no ODT, 1600-3200Mbps
DQS_40_3200   40 Ohm Data Strobe I/O with no ODT, 1600-3200Mbps
DQS_48_3200   48 Ohm Data Strobe I/O with no ODT, 1600-3200Mbps
DQS_IN_ODTOFF_3200 Data Strobe Input with no ODT, 1600-3200Mbps
DQS_IN_ODT34_3200  Data Strobe Input with 34ohm ODT, 1600-3200Mbps
DQS_IN_ODT40_3200  Data Strobe Input with 40ohm ODT, 1600-3200Mbps
DQS_IN_ODT48_3200  Data Strobe Input with 48ohm ODT, 1600-3200Mbps
DQS_IN_ODT60_3200  Data Strobe Input with 60ohm ODT, 1600-3200Mbps
DQS_IN_ODT80_3200  Data Strobe Input with 80ohm ODT, 1600-3200Mbps
DQS_IN_ODT120_3200 Data Strobe Input with 120ohm ODT, 1600-3200Mbps
DQS_IN_ODT240_3200 Data Strobe Input with 240ohm ODT, 1600-3200Mbps
[Model Selector] DM_DBI
DM_ODTOFF_3200   DM Input Model with no ODT, 1600-3200Mbps
DM_ODT34_3200   DM Input Model with 34ohm ODT, 1600-3200Mbps
DM_ODT40_3200   DM Input Model with 40ohm ODT, 1600-3200Mbps
DM_ODT48_3200   DM Input Model with 48ohm ODT, 1600-3200Mbps
DM_ODT60_3200   DM Input Model with 60ohm ODT, 1600-3200Mbps
DM_ODT80_3200   DM Input Model with 80ohm ODT, 1600-3200Mbps
DM_ODT120_3200   DM Input Model with 120ohm ODT, 1600-3200Mbps
DM_ODT240_3200   DM Input Model with 240ohm ODT, 1600-3200Mbps
DQ_34_3200   34 Ohm DBI I/O with no ODT, 1600-3200Mbps
DQ_40_3200   40 Ohm DBI I/O with no ODT, 1600-3200Mbps
DQ_48_3200   48 Ohm DBI I/O with no ODT, 1600-3200Mbps
DQ_IN_ODTOFF_3200  DBI Input with no ODT, 1600-3200Mbps
DQ_IN_ODT34_3200   DBI Input with 34ohm ODT, 1600-3200Mbps
DQ_IN_ODT40_3200   DBI Input with 40ohm ODT, 1600-3200Mbps
DQ_IN_ODT48_3200   DBI Input with 48ohm ODT, 1600-3200Mbps
DQ_IN_ODT60_3200   DBI Input with 60ohm ODT, 1600-3200Mbps
DQ_IN_ODT80_3200   DBI Input with 80ohm ODT, 1600-3200Mbps
DQ_IN_ODT120_3200  DBI Input with 120ohm ODT, 1600-3200Mbps
DQ_IN_ODT240_3200  DBI Input with 240ohm ODT, 1600-3200Mbps
NF_DQ   Non-Functioning DQ Terminator Model
[Model Selector] DM_DBI_TDQS
DM_ODTOFF_3200   DM Input Model with no ODT, 1600-3200Mbps
DM_ODT34_3200   DM Input Model with 34ohm ODT, 1600-3200Mbps
DM_ODT40_3200   DM Input Model with 40ohm ODT, 1600-3200Mbps
DM_ODT48_3200   DM Input Model with 48ohm ODT, 1600-3200Mbps
DM_ODT60_3200   DM Input Model with 60ohm ODT, 1600-3200Mbps
DM_ODT80_3200   DM Input Model with 80ohm ODT, 1600-3200Mbps
DM_ODT120_3200   DM Input Model with 120ohm ODT, 1600-3200Mbps
DM_ODT240_3200   DM Input Model with 240ohm ODT, 1600-3200Mbps
TDQS_ODT34_3200   TDQS Terminator Model with 34ohm ODT, 1600-3200Mbps
TDQS_ODT40_3200   TDQS Terminator Model with 40ohm ODT, 1600-3200Mbps
TDQS_ODT48_3200   TDQS Terminator Model with 48ohm ODT, 1600-3200Mbps
TDQS_ODT60_3200   TDQS Terminator Model with 60ohm ODT, 1600-3200Mbps
TDQS_ODT80_3200   TDQS Terminator Model with 80ohm ODT, 1600-3200Mbps
TDQS_ODT120_3200   TDQS Terminator Model with 120ohm ODT, 1600-3200Mbps
TDQS_ODT240_3200   TDQS Terminator Model with 240ohm ODT, 1600-3200Mbps
NF_DQ   Non-Functioning DQ Terminator Model
[Model Selector] TDQS
TDQS_ODTOFF_3200   TDQS Terminator Model with no ODT, 1600-3200Mbps
TDQS_ODT34_3200   TDQS Terminator Model with 34ohm ODT, 1600-3200Mbps
TDQS_ODT40_3200   TDQS Terminator Model with 40ohm ODT, 1600-3200Mbps
TDQS_ODT48_3200   TDQS Terminator Model with 48ohm ODT, 1600-3200Mbps
TDQS_ODT60_3200   TDQS Terminator Model with 60ohm ODT, 1600-3200Mbps
TDQS_ODT80_3200   TDQS Terminator Model with 80ohm ODT, 1600-3200Mbps
TDQS_ODT120_3200   TDQS Terminator Model with 120ohm ODT, 1600-3200Mbps
TDQS_ODT240_3200   TDQS Terminator Model with 240ohm ODT, 1600-3200Mbps
NF_DQ   Non-Functioning DQ Terminator Model
| Sparse Matrix Package Model for z32d_78ball_pkg (x4/x8)
[Define Package Model]  z32d_78ball_pkg
[Manufacturer]   Micron Technology, Inc.
[OEM]   Micron Technology, Inc.
[Description]   z22a package model for 78-ball x4/x8 FBGA
[Number of Pins]   52
[Pin Numbers]
L3  | A0
L7  | A1
M3  | A2
K7  | A3
K3  | A4
L8  | A5
L2  | A6
M8  | A7
M2  | A8
M7  | A9
J3  | A10
N2  | A11
J7  | A12
N8  | A13
N7  | A17
H3  | ACT#
L9  | ALERT#
K2  | BA0
K8  | BA1
J2  | BG0
J8  | BG1
H7  | CAS#
G3  | CKE
F8  | CK_C
F7  | CK_T
G7  | CS#
F3  | ODT
N3  | PARITY
H8  | RAS#
L1  | RESET#
H2  | WE#
C2  | DQ0
D3  | DQ2
D2  | DQ4
E3  | DQ6
B3  | DQS-C
C3  | DQS-T
A3  | TDQS-C
A7  | DM#
B7  | DQ1
D7  | DQ3
D8  | DQ5
E7  | DQ7
G9  | TEN
A1  | VDD
B2  | VDDQ_SUBNET_0
B8  | VDDQ_SUBNET_1
B1  | VPP-B1
M9  | VPP-M9
J1  | VREFCA
A9  | VSS
B9  | ZQ
[Model Data]
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[End Model Data]
[End Package Model]
| Sparse Matrix Package Model for z32d_96ball_pkg (x16)
[Define Package Model]  z32d_96ball_pkg
[Manufacturer]   Micron Technology, Inc.
[OEM]   Micron Technology, Inc.
[Description]   z32d package model for 96-ball x16 FBGA
[Number of Pins]   60
[Pin Numbers]
P3  | A0
P7  | A1
R3  | A2
N7  | A3
N3  | A4
P8  | A5
P2  | A6
R8  | A7
R2  | A8
R7  | A9
M3  | A10
T2  | A11
M7  | A12
T8  | A13
T7  | A17
L3  | ACT#
P9  | ALERT#
N2  | BA0
N8  | BA1
M2  | BG0
M8  | CAS#
K2  | CKE
K8  | CK_C
K7  | CK_T
L7  | CS#
K3  | ODT
T3  | PARITY
L8  | RAS#
P1  | RESET#
L2  | WE#
G2  | DQ0
F7  | DQ1
H3  | DQ2
H7  | DQ3
H2  | DQ4
H8  | DQ5
J3  | DQ6
J7  | DQ7
A3  | DQ8
B8  | DQ9
C3  | DQ10
C7  | DQ11
C2  | DQ12
C8  | DQ13
D3  | DQ14
D7  | DQ15
E7  | LDM#
F3  | LDQS-C
G3  | LDQS-T
E2  | UDM#
A7  | UDQS-C
B7  | UDQS-T
F9  | ZQ
N9  | TEN
B3  | VDD
A9  | VDDQ
B1  | VPP-B1
R9  | VPP-R9
M1  | VREFCA
B2  | VSS
[Model Data]
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[End Model Data]
[End Package Model]
| Models and submodels in the file (50): DQ_34_3200 (I/O), DQ_40_3200 (I/O), DQ_48_3200 (I/O), DQ_IN_ODTOFF_3200 (Input), DQ_IN_ODT34_3200 (Input), DQ_IN_ODT40_3200 (Input), DQ_IN_ODT48_3200 (Input), DQ_IN_ODT60_3200 (Input), DQ_IN_ODT80_3200 (Input), DQ_IN_ODT120_3200 (Input), DQ_IN_ODT240_3200 (Input), DQS_34_3200 (I/O), DQS_40_3200 (I/O), DQS_48_3200 (I/O), DQS_IN_ODTOFF_3200 (Input), DQS_IN_ODT34_3200 (Input), DQS_IN_ODT40_3200 (Input), DQS_IN_ODT48_3200 (Input), DQS_IN_ODT60_3200 (Input), DQS_IN_ODT80_3200 (Input), DQS_IN_ODT120_3200 (Input), DQS_IN_ODT240_3200 (Input), DM_ODTOFF_3200 (Input), DM_ODT34_3200 (Input), DM_ODT40_3200 (Input), DM_ODT48_3200 (Input), DM_ODT60_3200 (Input), DM_ODT80_3200 (Input), DM_ODT120_3200 (Input), DM_ODT240_3200 (Input), TDQS_ODTOFF_3200 (Terminator), TDQS_ODT34_3200 (Terminator), TDQS_ODT40_3200 (Terminator), TDQS_ODT48_3200 (Terminator), TDQS_ODT60_3200 (Terminator), TDQS_ODT80_3200 (Terminator), TDQS_ODT120_3200 (Terminator), TDQS_ODT240_3200 (Terminator), INPUT (Input), CLKIN (Input), ALERT (Open_sink), NF_DQ (Terminator), NF_INPUT (Terminator), 34ohm_ODT_3200 (Dynamic_clamp), 40ohm_ODT_3200 (Dynamic_clamp), 48ohm_ODT_3200 (Dynamic_clamp), 60ohm_ODT_3200 (Dynamic_clamp), 80ohm_ODT_3200 (Dynamic_clamp), 120ohm_ODT_3200 (Dynamic_clamp), 240ohm_ODT_3200 (Dynamic_clamp)
